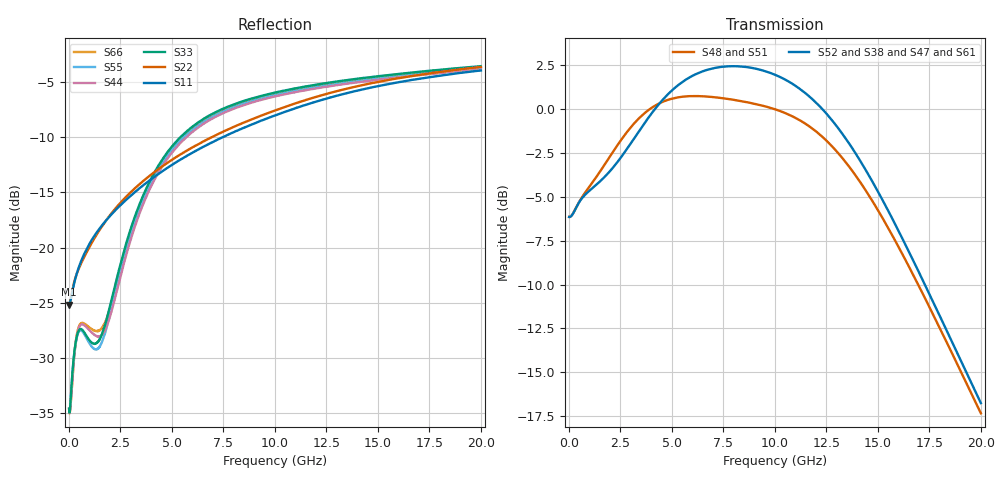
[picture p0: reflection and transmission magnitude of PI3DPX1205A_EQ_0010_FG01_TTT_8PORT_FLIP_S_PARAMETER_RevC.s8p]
! NPort=8 DATA=2000 NOISE=0 GROUPDELAY=0 COMPLEX_DATAFORMAT=POLAR
! NumOfBlock=1 NumOfParam=0
! .MODEL Smodel S TSTONEFILE=PI3DPX1205A_EQ_0010_FG01_TTT_8PORT_FLIP_S_PARAMETER_RevC.s8p TYPE=S
!  -- The above .MODEL line can be used for the S element in the netlist.
! The s parameter is extracted from the linear redriver, it is not bi-directional;
! only s(5,1)s(6,2)s(3,7)s(4,8) should be the insertion loss
!  Port definition:
!  Port1 = AIP
!  Port2 = AIN
!  Port3 = BOP
!  Port4 = BON
!  Port5 = AOP
!  Port6 = AON
!  Port7 = BIP
!  Port8 = BIN
# Hz S MA R  50
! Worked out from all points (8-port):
!   2000 points, 10 MHz to 20 GHz, reference 50 ohm
!   strongest paths, dB at 10 MHz, 5.01 GHz, 10.01 GHz, 15.01 GHz, 20 GHz:
!     S52: -6.1, 1.1, 2.0, -4.7, -16.8
!     S38: -6.1, 1.1, 1.9, -4.7, -16.8
!     S47: -6.1, 1.0, 2.0, -4.7, -16.7
!     S61: -6.1, 1.0, 1.9, -4.7, -16.7
!     S48: -6.1, 0.6, 0.0, -5.8, -17.3
!     S51: -6.1, 0.6, 0.0, -5.8, -17.3
!   lowest |S11| = -25.2 dB at 10 MHz (marker M1), VSWR 1.12, Z = 44.8 - j0.115 ohm
!   |S11| at or under -10 dB: start of sweep to 7.47 GHz
